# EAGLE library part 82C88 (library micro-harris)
MICROCONTROLLER/MEMORY DEVICE
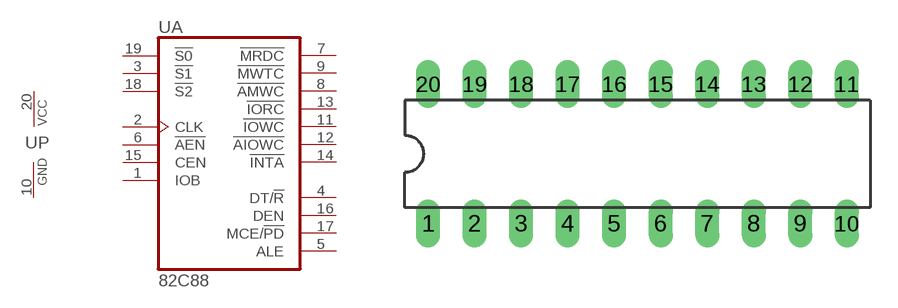
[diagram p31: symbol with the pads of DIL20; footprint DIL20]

Designator prefix U; gates A=82C88 P=PWRN

## 82C88 (MF: INTERSIL; MPN: CP82C88; OC_FARNELL: unknown; OC_NEWARK: 06F3294)  [DIL20]
1  A:IOB  in
2  A:CLK  in
3  A:!S1  in
4  A:DT/!R  out
5  A:ALE  out
6  A:!AEN  in
7  A:!MRDC  out
8  A:!AMWC  out
9  A:!MWTC  out
10  P:GND  pwr
11  A:!IOWC  out
12  A:!AIOWC  out
13  A:!IORC  out
14  A:!INTA  out
15  A:CEN  in
16  A:DEN  out
17  A:MCE/!PD  out
18  A:!S2  in
19  A:!S0  in
20  P:VCC  pwr

## Footprint DIL20 (pad centres in mm)
Dual In Line Package
drill 0.813 long: 1 -11.43,-3.81; 2 -8.89,-3.81; 3 -6.35,-3.81; 4 -3.81,-3.81; 5 -1.27,-3.81; 6 1.27,-3.81; 7 3.81,-3.81; 8 6.35,-3.81; 9 8.89,-3.81; 10 11.43,-3.81; 11 11.43,3.81; 12 8.89,3.81; 13 6.35,3.81; 14 3.81,3.81; 15 1.27,3.81; 16 -1.27,3.81; 17 -3.81,3.81; 18 -6.35,3.81; 19 -8.89,3.81; 20 -11.43,3.81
